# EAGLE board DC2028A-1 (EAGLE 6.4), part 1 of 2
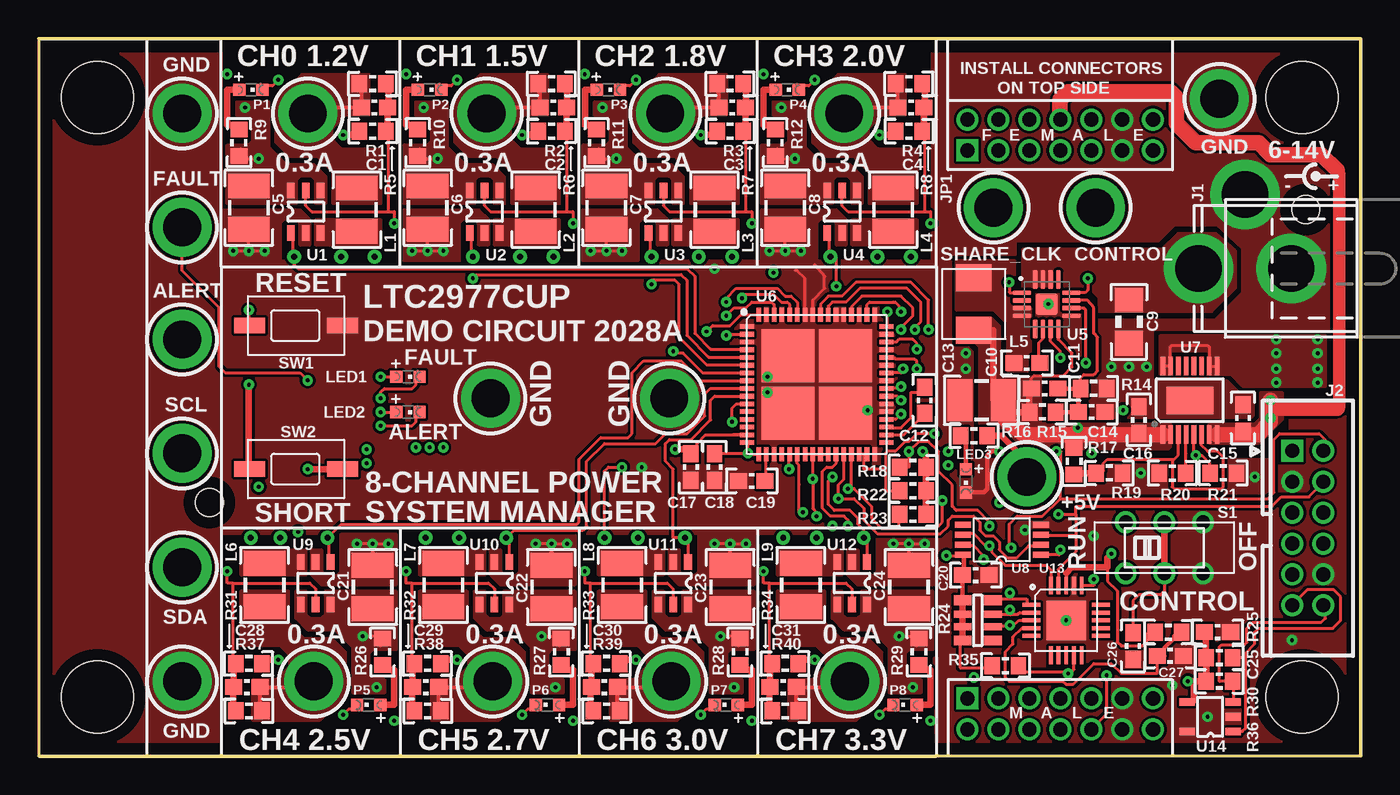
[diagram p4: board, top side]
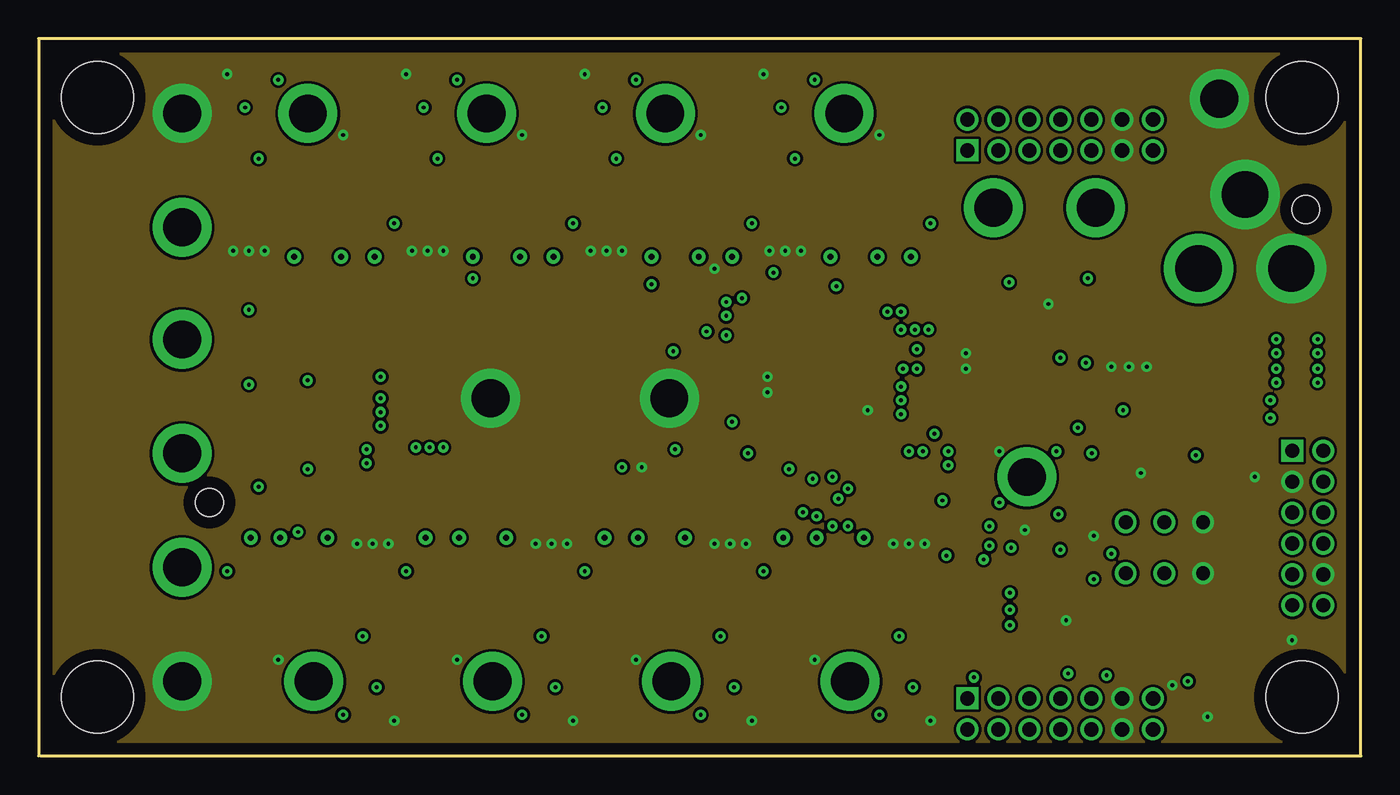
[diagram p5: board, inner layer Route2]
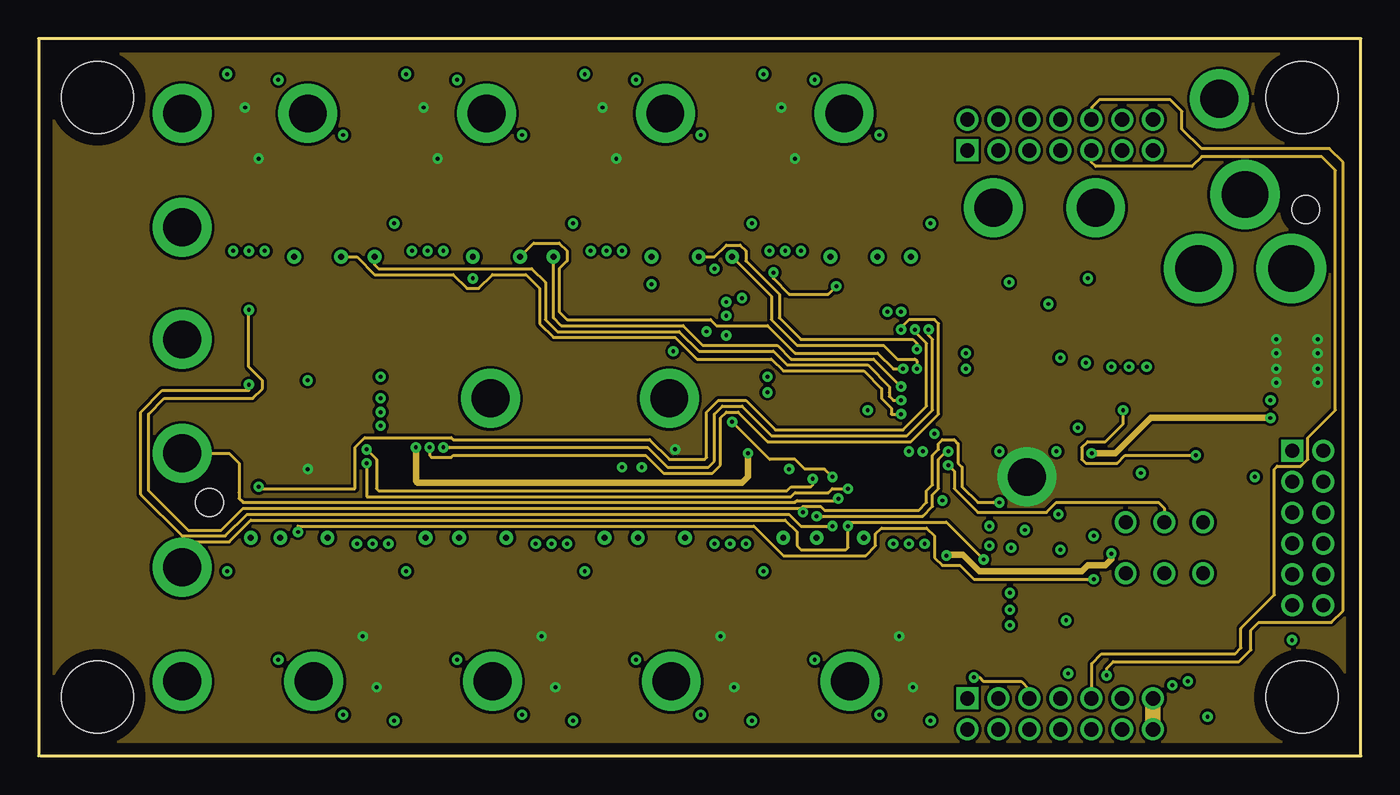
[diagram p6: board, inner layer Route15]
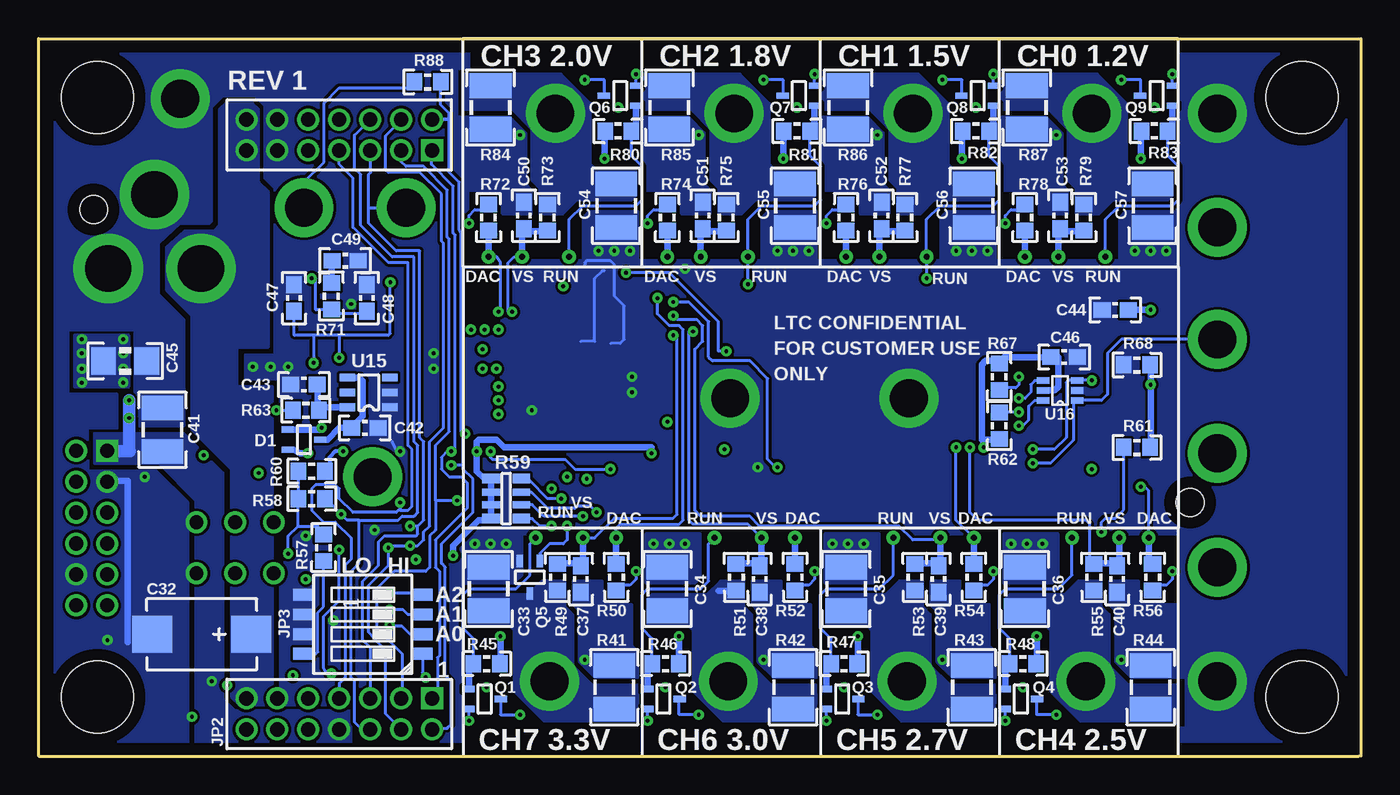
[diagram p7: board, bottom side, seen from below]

Size 85.47 x 46.35 mm. Coordinates in mm from the lower left corner, seen from the top.
Outline: 0,0 0,46.35 85.47,46.35 85.47,0 0.13,0
Copper layers (1*2+15*16): Top 0.035mm / dielectric 1.5mm / Route2 0.035mm / dielectric 0.15mm / Route15 0.035mm / dielectric 0.2mm / Bottom 0.035mm
Design rules: minimum track width 8mil, minimum drill 10mil, track to track 7mil, track to pad 7mil, pad to pad 7mil, via to via 7mil, smd to smd 4mil, copper to edge 30mil, drill to drill 15mil, minimum pad ring 10mil, minimum via ring 8mil, stop-mask expansion 4mil, vias tented up to drill 15mil, thermal gap 10mil
Holes 4.65 mm at 3.81,3.81 3.81,42.55 81.66,42.55 81.66,3.81
Holes 1.8 mm at 81.92,35.31 11.05,16.38

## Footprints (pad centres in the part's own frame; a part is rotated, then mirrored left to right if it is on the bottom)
C0603_BOX = smd 1.1 x 1: 1 -0.85,0; 2 0.85,0
C1210_BOX = smd 1.6 x 2.7: 1 -1.4,0; 2 1.4,0
C1206_BOX = smd 1.6 x 1.8: 1 -1.4,0; 2 1.4,0
C7343 = smd 2.6 x 2.4: + -3.2,0; - 3.2,0
SC70-3 = smd 0.4 x 0.8: 1 -0.65,-1.052; 2 0.65,-1.052; 3 0,1.052
PJ-002A = drill 3 pad 4.5: 1 -3,0; 2 0,-4.8; 3 3,0
CONN_DC1613 = drill 0.914 square: 1 -5,-1 | drill 0.914: 2 -5,1; 3 -3,-1; 4 -3,1; 5 -1,-1; 6 -1,1; 7 1,-1; 8 1,1; 9 3,-1; 10 3,1; 11 5,-1; 12 5,1
2X07M = drill 0.914 square: 1 -6,-1 | drill 0.914: 2 -6,1; 3 -4,-1; 4 -4,1; 5 -2,-1; 6 -2,1; 7 0,-1; 8 0,1; 9 2,-1; 10 2,1; 11 4,-1; 12 4,1; 13 6,-1; 14 6,1
SMT_DIP_4 = smd 1.27 x 0.762: 1 -3.861,1.905; 2 -3.861,0.635; 3 -3.861,-0.635; 4 -3.861,-1.905; 5 3.861,-1.905; 6 3.861,-0.635; 7 3.861,0.635; 8 3.861,1.905
L1210 = smd 1.6 x 2.7: 1 -1.4,0; 2 1.4,0
IHLP_1616AB = smd 1.75 x 2.3: 1 -1.7,0; 2 1.7,0
CHIPLED_0603 = smd 0.8 x 0.8: N 0,0.75; P 0,-0.75
R0603_BOX = smd 1 x 1.1: 1 -0.85,0; 2 0.85,0
R_VISHAY_CRA06S = smd 1.15 x 0.63: R1_1 -0.975,1.295; R1_2 0.975,1.295; R4_1 -0.975,-1.295; R4_2 0.975,-1.295 | smd 1.15 x 0.44: R2_1 -0.975,0.4; R2_2 0.975,0.4; R3_1 -0.975,-0.4; R3_2 0.975,-0.4
R1210_BOX = smd 1.6 x 2.7: 1 -1.4,0; 2 1.4,0
JS202011CQN = drill 0.9: 1 -2.5,1.65; 2 0,1.65; 3 2.5,1.65; 4 -2.5,-1.65; 5 0,-1.65; 6 2.5,-1.65
SWITCH_PTS635 = smd 2 x 1: SW1 -3,0; SW2 3,0
TP1 = drill 2.438 pad 3.81: TP 0,0
SOT-23-6 = smd 1 x 0.5: 1 -1.374,1.087; 2 -1.374,0.127; 3 -1.374,-0.833; 4 1.374,-0.833; 5 1.374,0.127; 6 1.374,1.087
QFN16_3X3 = smd 1.2 x 0.3: 1 -1.711,0.734; 2 -1.711,0.234; 3 -1.711,-0.266; 4 -1.711,-0.766; 9 1.489,-0.766; 10 1.489,-0.266; 11 1.489,0.234; 12 1.489,0.734 | smd 0.3 x 1.2: 5 -0.861,-1.616; 6 -0.361,-1.616; 7 0.139,-1.616; 8 0.639,-1.616; 13 0.639,1.584; 14 0.139,1.584; 15 -0.361,1.584; 16 -0.861,1.584 | smd 1.4 x 1.4: PAD -0.111,-0.016
QFN64_9X9 = smd 0.9 x 0.3: 1 -4.5,3.75; 2 -4.5,3.25; 3 -4.5,2.75; 4 -4.5,2.25; 5 -4.5,1.75; 6 -4.5,1.25; 7 -4.5,0.75; 8 -4.5,0.25; 9 -4.5,-0.25; 10 -4.5,-0.75; 11 -4.5,-1.25; 12 -4.5,-1.75; 13 -4.5,-2.25; 14 -4.5,-2.75; 15 -4.5,-3.25; 16 -4.5,-3.75; 33 4.5,-3.75; 34 4.5,-3.25; 35 4.5,-2.75; 36 4.5,-2.25; 37 4.5,-1.75; 38 4.5,-1.25; 39 4.5,-0.75; 40 4.5,-0.25; 41 4.5,0.25; 42 4.5,0.75; 43 4.5,1.25; 44 4.5,1.75; 45 4.5,2.25; 46 4.5,2.75; 47 4.5,3.25; 48 4.5,3.75 | smd 0.3 x 0.9: 17 -3.75,-4.5; 18 -3.25,-4.5; 19 -2.75,-4.5; 20 -2.25,-4.5; 21 -1.75,-4.5; 22 -1.25,-4.5; 23 -0.75,-4.5; 24 -0.25,-4.5; 25 0.25,-4.5; 26 0.75,-4.5; 27 1.25,-4.5; 28 1.75,-4.5; 29 2.25,-4.5; 30 2.75,-4.5; 31 3.25,-4.5; 32 3.75,-4.5; 49 3.75,4.5; 50 3.25,4.5; 51 2.75,4.5; 52 2.25,4.5; 53 1.75,4.5; 54 1.25,4.5; 55 0.75,4.5; 56 0.25,4.5; 57 -0.25,4.5; 58 -0.75,4.5; 59 -1.25,4.5; 60 -1.75,4.5; 61 -2.25,4.5; 62 -2.75,4.5; 63 -3.25,4.5; 64 -3.75,4.5 | smd 3.429 x 3.429: PAD1 -1.854,1.854; PAD2 1.854,1.854; PAD3 -1.854,-1.854; PAD4 1.854,-1.854
MSOP16_EXP = smd 1.2 x 0.3: 1 -2.213,1.75; 2 -2.213,1.25; 3 -2.213,0.75; 4 -2.213,0.25; 5 -2.213,-0.25; 6 -2.213,-0.75; 7 -2.213,-1.25; 8 -2.213,-1.75; 9 2.213,-1.75; 10 2.213,-1.25; 11 2.213,-0.75; 12 2.213,-0.25; 13 2.213,0.25; 14 2.213,0.75; 15 2.213,1.25; 16 2.213,1.75 | smd 1.778 x 3.048: EXP 0,0
MSOP-8 = smd 1.041 x 0.381: 1 -2.55,0.975; 2 -2.55,0.325; 3 -2.55,-0.325; 4 -2.55,-0.975; 5 2.479,-0.975; 6 2.479,-0.325; 7 2.479,0.325; 8 2.479,0.975
QFN20 = smd 1.143 x 0.254: 1 -2.25,1; 2 -2.25,0.5; 3 -2.25,0; 4 -2.25,-0.5; 5 -2.25,-1; 11 2.25,-1; 12 2.25,-0.5; 13 2.25,0; 14 2.25,0.5; 15 2.25,1 | smd 0.254 x 1.143: 6 -1,-2.25; 7 -0.5,-2.25; 8 0,-2.25; 9 0.5,-2.25; 10 1,-2.25; 16 1,2.25; 17 0.5,2.25; 18 0,2.25; 19 -0.5,2.25; 20 -1,2.25 | smd 2.54 x 2.54: PAD 0,0
SOT-23-5 = smd 1 x 0.5: 1 -1.649,0.95; 2 -1.649,0; 3 -1.649,-0.95; 4 1.333,-0.95; 5 1.333,0.95
SC70-6 = smd 0.4 x 0.8: 1 -0.65,-1.102; 2 0,-1.102; 3 0.65,-1.102; 4 0.65,1.102; 5 0,1.098; 6 -0.65,1.102
VIA = drill 0.381: 1 0,0

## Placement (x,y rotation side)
$$U$1  [LT_LOGO_LARGE_SM]  5.46,6.1 90 top
$$U$2  [LT_LOGO_LARGE_SM]  2.03,6.1 90 bottom
C1  220p  [C0603_BOX]  21.72,41.91 0 top
C2  220p  [C0603_BOX]  33.27,41.91 0 top
C3  220p  [C0603_BOX]  44.83,41.91 0 top
C4  220p  [C0603_BOX]  56.39,41.91 0 top
C5  10u/10V  [C1210_BOX]  13.59,35.43 270 top
C6  10u/10V  [C1210_BOX]  25.15,35.43 270 top
C7  10u/10V  [C1210_BOX]  36.7,35.43 270 top
C8  10u/10V  [C1210_BOX]  48.26,35.43 270 top
C9  10u/25V  [C1206_BOX]  70.48,28.07 90 top
C10  100n  [C0603_BOX]  63.88,25.4 0 top
C11  68p  [C0603_BOX]  65.02,23.75 0 top
C12  100n  [C0603_BOX]  57.28,22.99 270 top
C13  22u/10V  [C1210_BOX]  60.96,22.99 180 top
C14  47p  [C0603_BOX]  68.07,22.23 0 top
C15  1u  [C0603_BOX]  77.85,21.84 90 top
C16  1u  [C0603_BOX]  71.12,21.72 90 top
C17  1u  [C0603_BOX]  42.16,18.67 90 top
C18  100n  [C0603_BOX]  43.69,18.67 90 top
C19  100n  [C0603_BOX]  46.1,17.78 0 top
C20  100n  [C0603_BOX]  60.58,11.68 0 top
C21  10u/10V  [C1210_BOX]  21.59,10.92 90 top
C22  10u/10V  [C1210_BOX]  33.15,10.92 90 top
C23  10u/10V  [C1210_BOX]  44.7,10.92 90 top
C24  10u/10V  [C1210_BOX]  56.26,10.92 90 top
C25  1u  [C0603_BOX]  76.2,8 0 top
C26  1u  [C0603_BOX]  70.74,7.11 270 top
C27  1u  [C0603_BOX]  73.15,6.48 0 top
C28  220p  [C0603_BOX]  13.46,4.45 180 top
C29  220p  [C0603_BOX]  25.02,4.45 180 top
C30  220p  [C0603_BOX]  36.58,4.45 180 top
C31  220p  [C0603_BOX]  48.13,4.45 180 top
C32  47u/16V  [C7343]  74.93,7.87 180 bottom
C33  22u/10V  [C1210_BOX]  56.39,10.79 90 bottom
C34  22u/10V  [C1210_BOX]  44.83,10.79 90 bottom
C35  22u/10V  [C1210_BOX]  33.27,10.79 90 bottom
C36  22u/10V  [C1210_BOX]  21.72,10.79 90 bottom
C37  100n  [C0603_BOX]  50.42,11.43 90 bottom
C38  100n  [C0603_BOX]  38.86,11.43 90 bottom
C39  100n  [C0603_BOX]  27.3,11.43 90 bottom
C40  100n  [C0603_BOX]  15.75,11.43 90 bottom
C41  10u/10V  [C1210_BOX]  77.47,21.08 90 bottom
C42  1u  [C0603_BOX]  64.39,21.21 0 bottom
C43  4.7u  [C0603_BOX]  68.33,24 0 bottom
C44  10n  [C0603_BOX]  15.88,28.83 180 bottom
C45  10u/25V  [C1206_BOX]  79.88,25.53 0 bottom
C46  100n  [C0603_BOX]  19.18,25.78 0 bottom
C47  4.7u  [C0603_BOX]  68.96,29.59 90 bottom
C48  4.7p  [C0603_BOX]  64.26,29.59 90 bottom
C49  68p  [C0603_BOX]  65.66,32 0 bottom
C50  100n  [C0603_BOX]  54.1,34.92 270 bottom
C51  100n  [C0603_BOX]  42.55,34.92 270 bottom
C52  100n  [C0603_BOX]  30.99,34.92 270 bottom
C53  100n  [C0603_BOX]  19.43,34.92 270 bottom
C54  22u/10V  [C1210_BOX]  48.13,35.56 270 bottom
C55  22u/10V  [C1210_BOX]  36.58,35.56 270 bottom
C56  22u/10V  [C1210_BOX]  25.02,35.56 270 bottom
C57  22u/10V  [C1210_BOX]  13.46,35.56 270 bottom
D1  BAT30CWFILM  [SC70-3]  68.33,20.45 270 bottom
DRILEGEND  [DRILEGEND]  not placed on the board
J1  PJ-002A  [PJ-002A]  77.98,31.5 180 top
J2  CONN_DC1613  [CONN_DC1613]  82.04,14.73 270 top
JP1  FEMALE  [2X07M]  66.04,40.13 0 top
JP2  MALE  [2X07M]  66.04,2.72 180 bottom
JP3  TDA04H0SK1  [SMT_DIP_4]  64.52,8.51 0 bottom
L1  4.7uH  [L1210]  20.57,35.31 90 top
L2  4.7uH  [L1210]  32.13,35.31 90 top
L3  4.7uH  [L1210]  43.69,35.31 90 top
L4  4.7uH  [L1210]  55.24,35.31 90 top
L5  2.2uH  [IHLP_1616AB]  60.45,29.21 270 top
L6  4.7uH  [L1210]  14.61,11.05 270 top
L7  4.7uH  [L1210]  26.16,11.05 270 top
L8  4.7uH  [L1210]  37.72,11.05 270 top
L9  4.7uH  [L1210]  49.28,11.05 270 top
LED1  RED  [CHIPLED_0603]  23.88,24.51 270 top
LED2  RED  [CHIPLED_0603]  23.88,22.23 270 top
LED3  GREEN  [CHIPLED_0603]  59.94,17.78 180 top
P1  GREEN  [CHIPLED_0603]  13.72,43.05 270 top
P2  GREEN  [CHIPLED_0603]  25.27,43.05 270 top
P3  GREEN  [CHIPLED_0603]  36.83,43.05 270 top
P4  GREEN  [CHIPLED_0603]  48.39,43.05 270 top
P5  GREEN  [CHIPLED_0603]  21.34,3.3 90 top
P6  GREEN  [CHIPLED_0603]  32.89,3.3 90 top
P7  GREEN  [CHIPLED_0603]  44.45,3.3 90 top
P8  GREEN  [CHIPLED_0603]  56.01,3.3 90 top
Q1  SI1304  [SC70-3]  56.64,3.68 270 bottom
Q2  SI1304  [SC70-3]  45.09,3.68 270 bottom
Q3  SI1304  [SC70-3]  33.53,3.68 270 bottom
Q4  SI1304  [SC70-3]  21.97,3.68 270 bottom
Q5  SI1304  [SC70-3]  53.72,11.56 180 bottom
Q6  SI1304  [SC70-3]  47.88,42.67 90 bottom
Q7  SI1304  [SC70-3]  36.32,42.67 90 bottom
Q8  SI1304  [SC70-3]  24.77,42.67 90 bottom
Q9  SI1304  [SC70-3]  13.21,42.67 90 bottom
R1  100k  [R0603_BOX]  21.59,43.43 180 top
R2  100k  [R0603_BOX]  33.15,43.43 180 top
R3  100k  [R0603_BOX]  44.7,43.43 180 top
R4  100k  [R0603_BOX]  56.26,43.43 180 top
R5  200k  [R0603_BOX]  21.59,40.39 0 top
R6  115k  [R0603_BOX]  33.15,40.39 0 top
R7  80.6k  [R0603_BOX]  44.7,40.39 0 top
R8  66.5k  [R0603_BOX]  56.26,40.39 0 top
R9  3.01k  [R0603_BOX]  12.95,39.62 270 top
R10  3.01k  [R0603_BOX]  24.51,39.62 270 top
R11  3.01k  [R0603_BOX]  36.07,39.62 270 top
R12  3.01k  [R0603_BOX]  47.62,39.62 270 top
R14  10k  [R0603_BOX]  68.2,23.75 180 top
R15  73.2k  [R0603_BOX]  64.9,22.23 180 top
R16  3.01k  [R0603_BOX]  60.45,20.7 0 top
R17  46.4k  [R0603_BOX]  66.93,19.05 90 top
R18  10k  [R0603_BOX]  56.52,18.67 0 top
R19  10k  [R0603_BOX]  69.22,18.29 180 top
R20  249  [R0603_BOX]  73.28,18.29 0 top
R21  1.0k  [R0603_BOX]  76.58,18.29 180 top
R22  10k  [R0603_BOX]  56.52,17.14 0 top
R23  10k  [R0603_BOX]  56.52,15.62 0 top
R24  10k, 4X  [R_VISHAY_CRA06S]  60.71,8.76 180 top
R25  249  [R0603_BOX]  73.03,8 0 top
R26  3.01k  [R0603_BOX]  22.23,6.73 90 top
R27  3.01k  [R0603_BOX]  33.78,6.73 90 top
R28  3.01k  [R0603_BOX]  45.34,6.73 90 top
R29  3.01k  [R0603_BOX]  56.9,6.73 90 top
R30  10k  [R0603_BOX]  76.33,6.35 180 top
R31  47.5k  [R0603_BOX]  13.59,5.97 180 top
R32  42.2k  [R0603_BOX]  25.15,5.97 180 top
R33  36.5k  [R0603_BOX]  36.7,5.97 180 top
R34  32.4k  [R0603_BOX]  48.26,5.97 180 top
R35  10k  [R0603_BOX]  62.48,5.84 0 top
R36  10k  [R0603_BOX]  76.33,4.83 180 top
R37  100k  [R0603_BOX]  13.59,2.92 0 top
R38  100k  [R0603_BOX]  25.15,2.92 0 top
R39  100k  [R0603_BOX]  36.7,2.92 0 top
R40  100k  [R0603_BOX]  48.26,2.92 0 top
R41  470  [R1210_BOX]  48.26,4.45 270 bottom
R42  470  [R1210_BOX]  36.7,4.45 270 bottom
R43  470  [R1210_BOX]  25.15,4.45 270 bottom
R44  470  [R1210_BOX]  13.59,4.45 270 bottom
R45  100k  [R0603_BOX]  56.52,5.97 0 bottom
R46  100k  [R0603_BOX]  44.96,5.97 0 bottom
R47  100k  [R0603_BOX]  33.4,5.97 0 bottom
R48  100k  [R0603_BOX]  21.84,5.97 0 bottom
R49  100  [R0603_BOX]  51.94,11.56 90 bottom
R50  158k  [R0603_BOX]  48.13,11.56 90 bottom
R51  100  [R0603_BOX]  40.39,11.56 90 bottom
R52  174k  [R0603_BOX]  36.58,11.56 90 bottom
R53  100  [R0603_BOX]  28.83,11.56 90 bottom
R54  196k  [R0603_BOX]  25.02,11.56 90 bottom
R55  100  [R0603_BOX]  17.27,11.56 90 bottom
R56  210k  [R0603_BOX]  13.46,11.56 90 bottom
R57  10k  [R0603_BOX]  67.06,13.46 270 bottom
R58  10k  [R0603_BOX]  67.82,16.64 0 bottom
R59  10k, 4X  [R_VISHAY_CRA06S]  55.24,16.64 180 bottom
R60  10k  [R0603_BOX]  67.82,18.41 0 bottom
R61  OPT  [R0603_BOX]  14.48,19.94 0 bottom
R62  698  [R0603_BOX]  23.37,21.34 270 bottom
R63  2.49k  [R0603_BOX]  68.2,22.35 0 bottom
R67  698  [R0603_BOX]  23.37,24.51 270 bottom
R68  100k  [R0603_BOX]  14.48,25.27 0 bottom
R71  73.2k  [R0603_BOX]  66.55,29.72 270 bottom
R72  261k  [R0603_BOX]  56.39,34.8 270 bottom
R73  100  [R0603_BOX]  52.58,34.8 270 bottom
R74  294k  [R0603_BOX]  44.83,34.8 270 bottom
R75  100  [R0603_BOX]  41.02,34.8 270 bottom
R76  348k  [R0603_BOX]  33.27,34.8 270 bottom
R77  100  [R0603_BOX]  29.46,34.8 270 bottom
R78  442k  [R0603_BOX]  21.72,34.8 270 bottom
R79  100  [R0603_BOX]  17.91,34.8 270 bottom
R80  100k  [R0603_BOX]  48.01,40.39 180 bottom
R81  100k  [R0603_BOX]  36.45,40.39 180 bottom
R82  100k  [R0603_BOX]  24.89,40.39 180 bottom
R83  100k  [R0603_BOX]  13.34,40.39 180 bottom
R84  470  [R1210_BOX]  56.26,41.91 90 bottom
R85  470  [R1210_BOX]  44.7,41.91 90 bottom
R86  470  [R1210_BOX]  33.15,41.91 90 bottom
R87  470  [R1210_BOX]  21.59,41.91 90 bottom
R88  10k  [R0603_BOX]  60.33,43.56 0 bottom
S1  CONTROL  [JS202011CQN]  72.77,13.46 0 top
SW1  PTS635SL25SMTR LFS  [SWITCH_PTS635]  16.64,27.81 0 top
SW2  PTS635SK25SMTR LFS  [SWITCH_PTS635]  16.64,18.54 0 top
TP1  TESTPOINT_BIG  [TP1]  76.33,42.47 0 top
TP2  TESTPOINT_BIG  [TP1]  9.27,41.53 0 top
TP3  TESTPOINT_BIG  [TP1]  17.4,41.53 90 top
TP4  TESTPOINT_BIG  [TP1]  28.96,41.53 90 top
TP5  TESTPOINT_BIG  [TP1]  40.51,41.53 90 top
TP6  TESTPOINT_BIG  [TP1]  52.07,41.53 90 top
TP7  TESTPOINT_BIG  [TP1]  61.72,35.43 0 top
TP8  TESTPOINT_BIG  [TP1]  68.33,35.43 0 top
TP9  TESTPOINT_BIG  [TP1]  9.27,34.16 0 top
TP10  TESTPOINT_BIG  [TP1]  9.27,26.92 0 top
TP11  TESTPOINT_BIG  [TP1]  40.77,23.11 0 top
TP12  TESTPOINT_BIG  [TP1]  29.21,23.11 0 top
TP13  TESTPOINT_BIG  [TP1]  9.27,19.56 0 top
TP14  TESTPOINT_BIG  [TP1]  63.88,18.03 0 top
TP15  TESTPOINT_BIG  [TP1]  9.27,12.19 0 top
TP16  TESTPOINT_BIG  [TP1]  9.27,4.83 0 top
TP17  TESTPOINT_BIG  [TP1]  17.78,4.83 270 top
TP18  TESTPOINT_BIG  [TP1]  29.34,4.83 270 top
TP19  TESTPOINT_BIG  [TP1]  40.89,4.83 270 top
TP20  TESTPOINT_BIG  [TP1]  52.45,4.83 270 top
U1  LTC3405AES6  [SOT-23-6]  17.4,35.18 90 top
U2  LTC3405AES6  [SOT-23-6]  28.96,35.18 90 top
U3  LTC3405AES6  [SOT-23-6]  40.51,35.18 90 top
U4  LTC3405AES6  [SOT-23-6]  52.07,35.18 90 top
U5  LTC3604IUD  [QFN16_3X3]  65.28,29.21 0 top
U6  LTC2977CUP  [QFN64_9X9]  50.29,24 0 top
U7  LTC4415IMSE  [MSOP16_EXP]  74.42,22.99 90 top
U8  LTC4313CMS8  [MSOP-8]  62.23,13.97 180 top
U9  LTC3405AES6  [SOT-23-6]  17.78,11.18 270 top
U10  LTC3405AES6  [SOT-23-6]  29.34,11.18 270 top
U11  LTC3405AES6  [SOT-23-6]  40.89,11.18 270 top
U12  LTC3405AES6  [SOT-23-6]  52.45,11.18 270 top
U13  MCP23008-E/ML  [QFN20]  66.42,8.76 0 top
U14  24AA02T-I/OT  [SOT-23-5]  75.56,2.54 180 top
U15  LT6654BMPS6-1.25  [SOT-23-6]  64.14,23.62 180 bottom
U16  SN74LVC2G34DCK  [SC70-6]  19.43,23.62 90 bottom
U$8  [DC2028_FRAME]  not placed on the board
VSNSN1  TESPOINT_SMD  [VIA]  16.51,32.26 180 top
VSNSN2  TESPOINT_SMD  [VIA]  28.07,32.26 180 top
VSNSN3  TESPOINT_SMD  [VIA]  39.62,32.26 180 top
VSNSN4  TESPOINT_SMD  [VIA]  51.18,32.26 180 top
VSNSN5  TESPOINT_SMD  [VIA]  18.67,14.1 0 top
VSNSN6  TESPOINT_SMD  [VIA]  30.23,14.1 0 top
VSNSN7  TESPOINT_SMD  [VIA]  41.78,14.1 0 top
VSNSN8  TESPOINT_SMD  [VIA]  53.34,14.1 0 top
VSNSN9  TESPOINT_SMD  [VIA]  50.29,14.1 0 bottom
VSNSN10  TESPOINT_SMD  [VIA]  48.13,14.1 0 bottom
VSNSN11  TESPOINT_SMD  [VIA]  38.73,14.1 0 bottom
VSNSN12  TESPOINT_SMD  [VIA]  36.58,14.1 0 bottom
VSNSN13  TESPOINT_SMD  [VIA]  27.18,14.1 0 bottom
VSNSN14  TESPOINT_SMD  [VIA]  25.02,14.1 0 bottom
VSNSN15  TESPOINT_SMD  [VIA]  15.62,14.1 0 bottom
VSNSN16  TESPOINT_SMD  [VIA]  13.72,14.1 0 bottom
VSNSN17  TESPOINT_SMD  [VIA]  56.39,32.26 180 bottom
VSNSN18  TESPOINT_SMD  [VIA]  54.23,32.26 180 bottom
VSNSN19  TESPOINT_SMD  [VIA]  44.83,32.26 180 bottom
VSNSN20  TESPOINT_SMD  [VIA]  42.67,32.26 180 bottom
VSNSN21  TESPOINT_SMD  [VIA]  33.27,32.26 180 bottom
VSNSN22  TESPOINT_SMD  [VIA]  31.11,32.26 180 bottom
VSNSN23  TESPOINT_SMD  [VIA]  21.72,32.26 180 bottom
VSNSN24  TESPOINT_SMD  [VIA]  19.56,32.26 180 bottom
